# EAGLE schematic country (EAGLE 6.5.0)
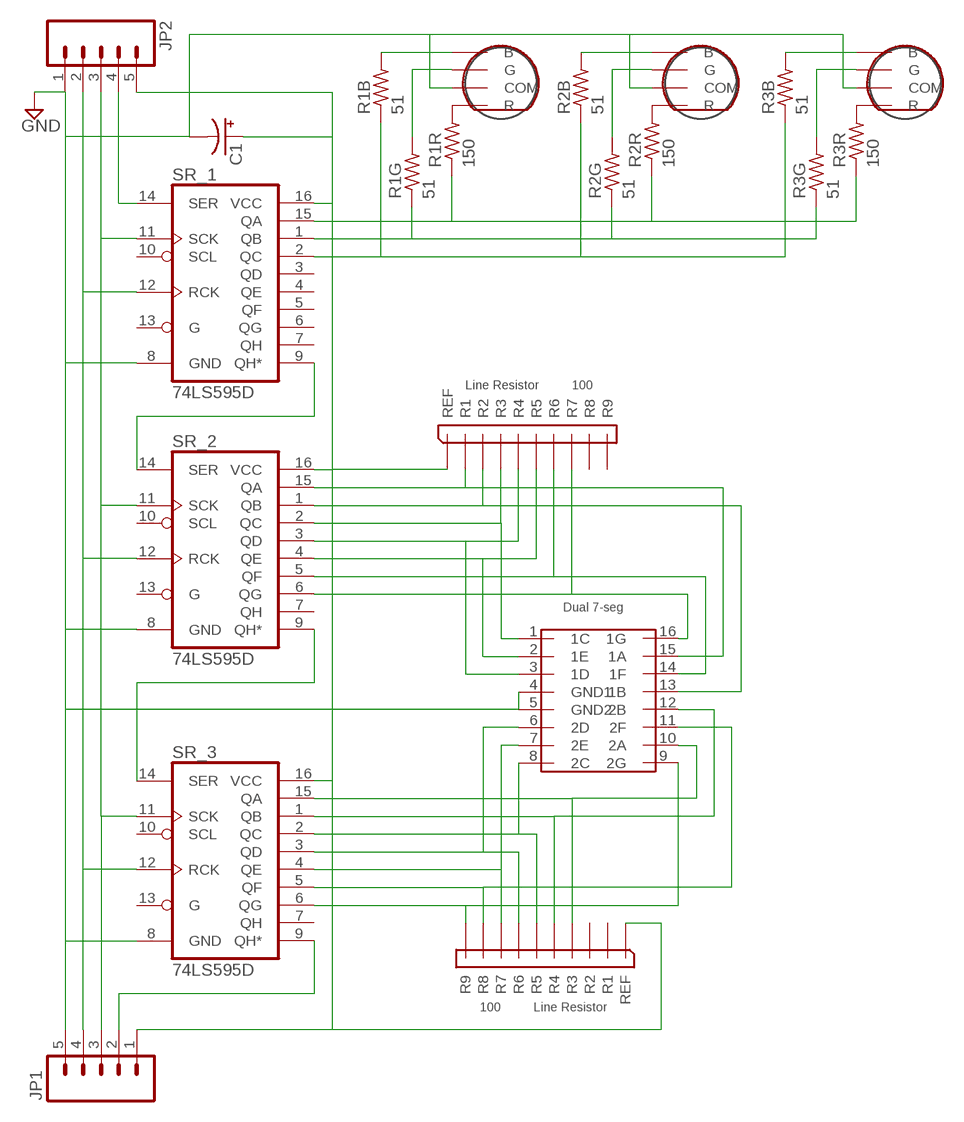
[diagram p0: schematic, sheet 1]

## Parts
C1  CPOL-USE2,5-6E  [E2,5-6E]
JP1  M05LOCK  [1X05_LOCK]
JP2  M05LOCK  [1X05_LOCK]
R1B  51  R-US_0204/5  [0204/5]
R1G  51  R-US_0204/5  [0204/5]
R1R  150  R-US_0204/5  [0204/5]
R2B  51  R-US_0204/5  [0204/5]
R2G  51  R-US_0204/5  [0204/5]
R2R  150  R-US_0204/5  [0204/5]
R3B  51  R-US_0204/5  [0204/5]
R3G  51  R-US_0204/5  [0204/5]
R3R  150  R-US_0204/5  [0204/5]
SR_1  74LS595D  [SO16]
SR_2  74LS595D  [SO16]
SR_3  74LS595D  [SO16]
U$1  HDSP-G03E  [HDSP-G]
U$2  100  4610X  [4610X]
U$3  100  4610X  [4610X]
U$4  RGBLED  [3LED]
U$5  RGBLED  [3LED]
U$6  RGBLED  [3LED]

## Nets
GND: C1.- JP1.5 JP2.1 SR_1.8(GND) SR_2.8(GND) SR_3.8(GND) U$1.4(GND1) U$1.5(GND2) U$4.COM U$5.COM U$6.COM
N$1: SR_1.9(QH*) SR_2.14(SER)
N$2: SR_2.9(QH*) SR_3.14(SER)
N$3: C1.+ JP1.1 JP2.5 SR_1.16(VCC) SR_2.16(VCC) SR_3.16(VCC) U$2.REF U$3.REF
N$4: SR_2.15(QA) U$1.15(1A) U$2.R1
N$5: SR_2.1(QB) U$1.13(1B) U$2.R2
N$6: SR_2.2(QC) U$1.1(1C) U$2.R3
N$7: SR_2.3(QD) U$1.3(1D) U$2.R4
N$8: R1R.2 U$4.R
N$9: SR_2.5(QF) U$1.14(1F) U$2.R6
N$10: SR_2.6(QG) U$1.16(1G) U$2.R7
N$11: SR_3.6(QG) U$1.9(2G) U$3.R9
N$12: SR_3.5(QF) U$1.11(2F) U$3.R8
N$13: SR_3.4(QE) U$1.7(2E) U$3.R7
N$14: SR_3.3(QD) U$1.6(2D) U$3.R6
N$15: SR_3.2(QC) U$1.8(2C) U$3.R5
N$16: SR_2.4(QE) U$1.2(1E) U$2.R5
N$17: SR_3.15(QA) U$1.10(2A) U$3.R3
N$18: R2R.2 U$5.R
N$19: SR_3.1(QB) U$1.12(2B) U$3.R4
N$20: R3R.2 U$6.R
N$21: JP1.4 JP2.2 SR_1.12(RCK) SR_2.12(RCK) SR_3.12(RCK)
N$22: JP1.3 JP2.3 SR_1.11(SCK) SR_2.11(SCK) SR_3.11(SCK)
N$23: JP2.4 SR_1.14(SER)
N$24: JP1.2 SR_3.9(QH*)
N$25: R1G.2 U$4.G
N$26: R2G.2 U$5.G
N$27: R3G.2 U$6.G
N$28: R1B.2 U$4.B
N$29: R2B.2 U$5.B
N$30: R3B.2 U$6.B
N$31: R1R.1 R2R.1 R3R.1 SR_1.15(QA)
N$32: R1G.1 R2G.1 R3G.1 SR_1.1(QB)
N$33: R1B.1 R2B.1 R3B.1 SR_1.2(QC)
Unconnected: SR_1.3(QD) SR_1.4(QE) SR_1.5(QF) SR_1.6(QG) SR_1.7(QH) SR_1.10(SCL) SR_1.13(G) SR_2.7(QH) SR_2.10(SCL) SR_2.13(G) SR_3.7(QH) SR_3.10(SCL) SR_3.13(G) U$2.R8 U$2.R9 U$3.R1 U$3.R2

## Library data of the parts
C1 = Power Supply:CPOL-US: POLARIZED CAPACITOR, American symbol
JP1 JP2 = SparkFun-Connectors:M05: Header 5 Standard 5-pin 0.1" header. Use with straight break away headers (SKU : PRT-00116), right angle break away headers (PRT-00553), swiss pins (PRT-00743), machine pins (PRT-00117), and female headers (PRT-00115). Molex polarized connector foot print use with SKU : PRT-08230 with associated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
R1B R1G R1R R2B R2G R2R R3B R3G R3R = resistor:R-US_: RESISTOR, American symbol
SR_1-SR_3 = SparkFun-DigitalIC:74*595: 8-bit SHIFT REGISTER, output latch; PROD_ID: IC-07875
U$1 = RISK:HDSP-G03E
U$2 U$3 = RISK:4610X
U$4-U$6 = RISK:RGBLED

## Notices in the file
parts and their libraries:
SparkFun-DigitalIC: Licensing: Creative Commons ShareAlike 4.0 International - https://creativecommons.org/licenses/by-sa/4.0
